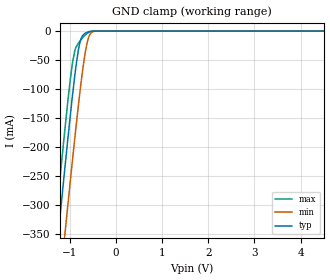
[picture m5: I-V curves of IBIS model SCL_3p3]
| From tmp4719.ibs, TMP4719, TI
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|   Model
[Model]   SCL_3p3
Model_type   Input
Vinl = .99
Vinh = 2.31
|   typ   min   max
C_comp   1.34pF   1.32pF   1.35pF
[Voltage Range]   3.3   2.7   3.6
[Temperature Range]   25   125   -40
[Power Clamp Reference]   3.3   2.7   3.6
[GND Clamp Reference]   0   0   0
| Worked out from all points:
|   GND clamp passes 1 mA (typ) near -0.58 V on its own axis
[GND Clamp]
|   Voltage   I(typ)   I(min)   I(max)
-3.3V     -2.077A    -2.182A    -2.02A
-1.379V   -458.1mA   -572.6mA   -391.8mA
-1.211V   -321.1mA   -436mA     -254.4mA
-1.102V   -234.4mA   -349mA     -168.2mA
-1.092V   -226.6mA   -341.1mA   -160.6mA
-993.3mV  -150.5mA   -263.6mA   -88mA
-894.3mV  -79.88mA   -188.2mA   -35.59mA
-775.5mV  -18.9mA    -103.2mA   -17.04mA
-627mV    -2.193mA   -21.72mA   -4.275mA
-547.8mV  -486.9uA   -4.124mA   -939uA
-419.1mV  -10.31uA   -127.6uA   -8.323uA
6.6V      0A         0A         0A
